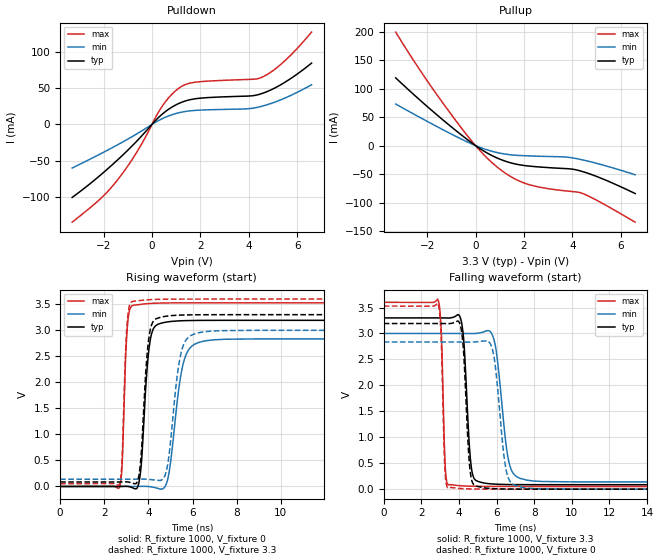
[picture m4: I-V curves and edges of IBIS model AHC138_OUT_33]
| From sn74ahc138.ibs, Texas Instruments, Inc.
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[Model]   AHC138_OUT_33
Model_type  Output
Vref =   0
Rref =   1000
Cref =   15p
Vmeas =   1.65
| variable   typ   min   max
C_comp   3.26pF   2.42pF   4.28pF
| C_pullup   3.41pF   2.43pF   4.28pF
| C_pulldown   3.11pF   2.42pF   3.86pF
[Temperature Range]   40   100   -40
| Ambient temperature   25   85   -40
[Voltage range]   3.3   3   3.6
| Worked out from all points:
|   slope of the pulldown table from 0 to 0.495 V, typ, clamps not added: 30.8 ohm
|   slope of the pullup table from 0 to 0.495 V, typ, clamps not added: 37.1 ohm
|   rising waveform, R_fixture 1000, V_fixture 0: 20-80 % time 289ps typ, 496ps min, 173ps max; typ from 0 V to 3.19 V
|   falling waveform, R_fixture 1000, V_fixture 3.3: 20-80 % time 281ps typ, 498ps min, 159ps max; typ from 3.3 V to 0.086 V
|   rising waveform, R_fixture 1000, V_fixture 3.3: 20-80 % time 277ps typ, 451ps min, 169ps max; typ from 0.086 V to 3.3 V
|   falling waveform, R_fixture 1000, V_fixture 0: 20-80 % time 265ps typ, 453ps min, 153ps max; typ from 3.19 V to 0 V
[Pulldown]
| AHC138_OUT_33
|   Voltage   I(typ)   I(min)   I(max)
-3.3V     -100.7mA   -60.13mA   -134.8mA
-2.14V    -70.19mA   -40.8mA    -102.8mA
-1.435V   -49.38mA   -28.35mA   -77.03mA
-600mV    -22.1mA    -12.49mA   -36.8mA
395mV     13.29mA    7.442mA    23.56mA
1.04V     27.78mA    15.47mA    48.12mA
1.365V    32.17mA    17.78mA    54.77mA
1.745V    35.15mA    19.25mA    58mA
3.935V    39.06mA    21.56mA    62mA
4.54V     42.55mA    25.05mA    65mA
5.44V     56.97mA    35.53mA    86.11mA
6.6V      84.58mA    54.72mA    127.3mA
[Pullup]
| AHC138_OUT_33
|   Voltage   I(typ)   I(min)   I(max)
-3.3V     118.9mA    72.92mA    199.3mA
-2.04V    70.24mA    43.48mA    116.4mA
-630mV    20.24mA    12.36mA    33.38mA
205mV     -5.911mA   -3.486mA   -9.804mA
950mV     -22.84mA   -12.77mA   -39.56mA
1.57V     -31.55mA   -16.65mA   -57.16mA
2.195V    -35.88mA   -18.08mA   -68.3mA
2.815V    -38.12mA   -18.92mA   -74.28mA
3.68V     -40.3mA    -19.96mA   -79.3mA
4.25V     -43.54mA   -23.54mA   -81.94mA
4.95V     -53.28mA   -30.54mA   -94.61mA
6.6V      -84.2mA    -51.23mA   -134.5mA
[Ramp]
| AHC138_OUT_33
| variable   typ   min   max
dV/dt_r   1.94/3.05E-10   1.73/5.08E-10   2.14/1.86E-10
dV/dt_f   1.97/3.00E-10   1.75/5.08E-10   2.17/1.72E-10
R_load = 1000
[Rising Waveform]
| AHC138_OUT_33
R_fixture =   1000
C_fixture =   0
L_fixture =   0
V_fixture =   0
V_fixture_min = 0
V_fixture_max = 0
|   Time   V(typ)   V(min)   V(max)
0s        185.5pV    439pV      70.39pV
2.71ns    -119.2uV   9.024uV    4.944mV
3.045ns   2.131mV    -145.8uV   3.055V
3.345ns   -38.01mV   -70.58uV   3.484V
3.66ns    339.4mV    2.043mV    3.499V
4.105ns   2.861V     -6.114mV   3.516V
4.81ns    3.157V     47.88mV    3.525V
5.615ns   3.185V     2.42V      3.527V
6.67ns    3.191V     2.803V     3.528V
50ns      3.192V     2.835V     3.528V
[Falling Waveform]
| AHC138_OUT_33
R_fixture =   1000
C_fixture =   0
L_fixture =   0
V_fixture =   3.3
V_fixture_min = 3
V_fixture_max = 3.6
|   Time   V(typ)   V(min)   V(max)
0s        3.3V       3V         3.6V
2.9ns     3.3V       3V         3.637V
3.275ns   3.299V     3V         409.9mV
3.47ns    3.298V     3V         81.59mV
4.135ns   3.217V     3V         64.38mV
4.665ns   399.4mV    2.998V     56.72mV
5.32ns    119.3mV    3.033V     53.67mV
6.705ns   88.9mV     450mV      52.38mV
7.6ns     86.78mV    173.6mV    52.26mV
50ns      86.09mV    139.4mV    52.22mV
[Rising Waveform]
| AHC138_OUT_33
R_fixture =   1000
C_fixture =   0
L_fixture =   0
V_fixture =   3.3
V_fixture_min = 3
V_fixture_max = 3.6
|   Time   V(typ)   V(min)   V(max)
0s        86.09mV    139.4mV    52.22mV
2.7ns     85.96mV    139.4mV    54.82mV
3.04ns    87.66mV    139.3mV    3.155V
3.335ns   56.09mV    139.4mV    3.56V
3.625ns   385.7mV    140.9mV    3.572V
4.055ns   2.943V     134.7mV    3.588V
4.725ns   3.265V     184.9mV    3.597V
5.51ns    3.293V     2.614V     3.599V
6.48ns    3.299V     2.969V     3.6V
50ns      3.3V       3V         3.6V
[Falling Waveform]
| AHC138_OUT_33
R_fixture =   1000
C_fixture =   0
L_fixture =   0
V_fixture =   0
V_fixture_min = 0
V_fixture_max = 0
|   Time   V(typ)   V(min)   V(max)
0s        3.192V     2.835V     3.528V
2.895ns   3.192V     2.835V     3.56V
3.395ns   3.19V      2.835V     28.41mV
4.105ns   3.108V     2.835V     11.75mV
4.605ns   319.4mV    2.835V     4.607mV
5.23ns    31.61mV    2.852V     1.562mV
5.855ns   9.458mV    2.569V     571.2uV
6.57ns    2.832mV    273.3mV    191.1uV
7.385ns   797.7uV    32.62mV    57.1uV
50ns      3.985nV    380.1pV    -4.01nV
